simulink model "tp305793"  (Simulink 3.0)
settings: Solver=ode45  StartTime=0.0  StopTime=10  RelTol=1e-3

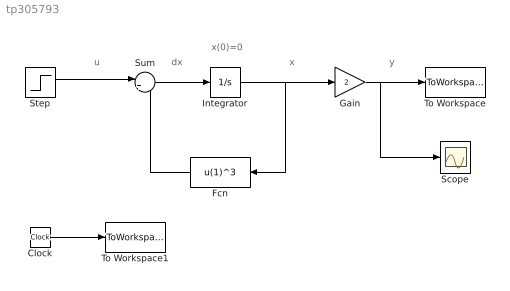
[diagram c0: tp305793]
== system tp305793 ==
  note: dx
  note: x
  note: y
  note: x(0)=0
  note: u
  Clock : Clock
  Fcn : Fcn  Orientation=left  Expr=u(1)^3
  Gain : Gain  Gain=2  SaturateOnIntegerOverflow=on
  Integrator : Integrator  ExternalReset=none  InitialConditionSource=internal  InitialCondition=0  LimitOutput=off  UpperSaturationLimit=inf  LowerSaturationLimit=-inf  ShowSaturationPort=off  ShowStatePort=off  AbsoluteTolerance=auto
  Scope : Scope
  Step : Step  Time=1  Before=0  After=1  SampleTime=0
  Sum : Sum  Inputs=|+-  SaturateOnIntegerOverflow=on
  To Workspace : ToWorkspace  VariableName=y  SampleTime=-1  SaveFormat=Matrix
  To Workspace1 : ToWorkspace  VariableName=t  SampleTime=-1  SaveFormat=Matrix
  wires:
  Integrator/1 -> Gain/1, Fcn/1
  Sum/1 -> Integrator/1
  Gain/1 -> To Workspace/1, Scope/1
  Fcn/1 -> Sum/2
  Clock/1 -> To Workspace1/1
  Step/1 -> Sum/1
